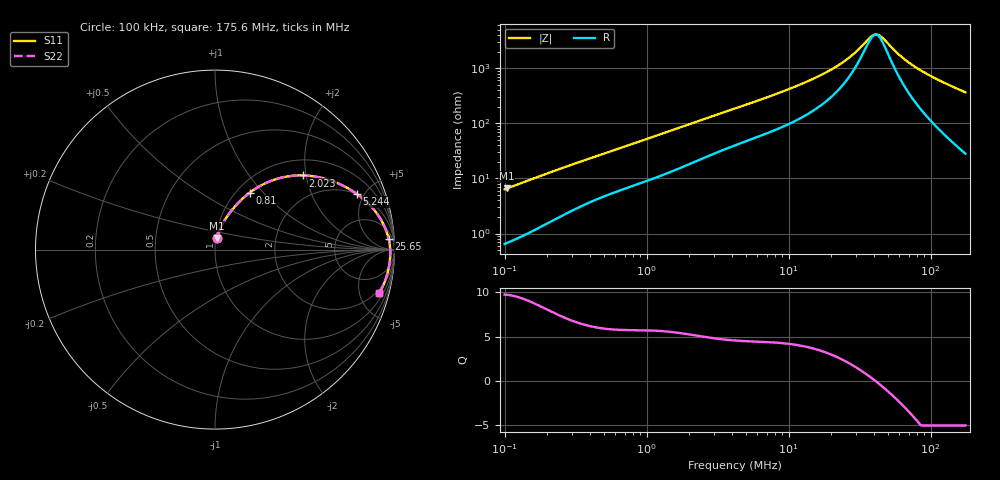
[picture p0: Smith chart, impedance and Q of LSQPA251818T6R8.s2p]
! LSQPA251818T6R8  S-PARAMETER MODEL  ( General Type )
! Model Generated by TAIYO YUDEN Corporation (http://www.ty-top.com)
! Version 3.0
! TAIYO YUDEN Control No. 160907NF25SB-FKC
! Copyright(c) 2007 TAIYO YUDEN CO.,LTD. All Rights Reserved.
! Product Description (link to TY-COMPAS)
! https://ds.yuden.co.jp/TYCOMPAS/or/detail?pn=LSQPA251818T6R8M&u=M
! Products Name : Inductors
! Characteristics :
!  Inductance : 6.8 uH , SRF(min) : 38 MHz , DC Resistance(max) : 0.39 Ohm
!  Rated Current : Saturation :550 mA , Temp Rise : 740 mA (40 degC)
!  Case Size : 2.5 x 1.8 / 0.098 x 0.071 [mm/inch] , Thickness : 1.8 / 0.071 [mm/inch]
!  (Conditions: Temperature = 25 degC , DC Bias Current/Voltage = 0A / 0V)
! External Node Assignments :
!  1  o---GGG---o  2
! GND o---------o GND
! Frequency Range : 0.1MHz  -  175.64884MHz  [ 402 STEP ]
# MHz S RI R 50
! Freq[MHz].  S11 Real  S11 Imag  S21 Real  S21 Imag  S12 Real  S12 Imag  S22 Real  S22 Imag
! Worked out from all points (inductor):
!   401 points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, 100 kHz to 175.6 MHz, reference 50 ohm
!   read as one part in series: L = 9.96 uH near 103.8 kHz
!   highest Q = 9.7 at 103.8 kHz (marker M1), where L = 10 uH
!   self-resonance near 40.89 MHz
!   S11 on the Smith chart (normalised r, x): 100 kHz: 1.01, +0.13; 810 kHz: 1.15, +0.85; 2.023 MHz: 1.37, +1.92; 5.244 MHz: 1.99, +4.41; 25.65 MHz: 13, +26; 175.6 MHz: 1.56, -7.28
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0.1  0.0103 0.062  0.9897 -0.062  0.9897 -0.062  0.0103 0.062
0.103806  0.0109 0.0642  0.9891 -0.0642  0.9891 -0.0642  0.0109 0.0642
0.349525  0.0668 0.1836  0.9332 -0.1836  0.9332 -0.1836  0.0668 0.1836
0.547213  0.1206 0.2509  0.8794 -0.2509  0.8794 -0.2509  0.1206 0.2509
0.810029  0.1941 0.3176  0.8059 -0.3176  0.8059 -0.3176  0.1941 0.3176
1.221676  0.3084 0.3816  0.6916 -0.3816  0.6916 -0.3816  0.3084 0.3816
2.022878  0.491 0.4132  0.509 -0.4132  0.509 -0.4132  0.491 0.4132
4.270063  0.7382 0.3431  0.2618 -0.3431  0.2618 -0.3431  0.7382 0.3431
5.243992  0.7896 0.3107  0.2104 -0.3107  0.2104 -0.3107  0.7896 0.3107
9.01361  0.8892 0.2178  0.1108 -0.2178  0.1108 -0.2178  0.8892 0.2178
14.64875  0.9398 0.1383  0.0602 -0.1383  0.0602 -0.1383  0.9398 0.1383
20.12325  0.9586 0.092  0.0414 -0.092  0.0414 -0.092  0.9586 0.092
25.65365  0.9678 0.0593  0.0322 -0.0593  0.0322 -0.0593  0.9678 0.0593
29.78805  0.9717 0.04  0.0283 -0.04  0.0283 -0.04  0.9717 0.04
37.27189  0.9753 0.0117  0.0247 -0.0117  0.0247 -0.0117  0.9753 0.0117
40.16316  0.976 0.00227  0.024 -0.00227  0.024 -0.00227  0.976 0.00227
44.09465  0.9765 -0.00958  0.0235 0.00958  0.0235 0.00958  0.9765 -0.00958
51.20104  0.9765 -0.0289  0.0235 0.0289  0.0235 0.0289  0.9765 -0.0289
64.06461  0.9746 -0.0592  0.0254 0.0592  0.0254 0.0592  0.9746 -0.0592
83.211  0.9689 -0.0982  0.0311 0.0982  0.0311 0.0982  0.9689 -0.0982
118.6592  0.9523 -0.1602  0.0477 0.1602  0.0477 0.1602  0.9523 -0.1602
175.6488  0.914 -0.2445  0.086 0.2445  0.086 0.2445  0.914 -0.2445
